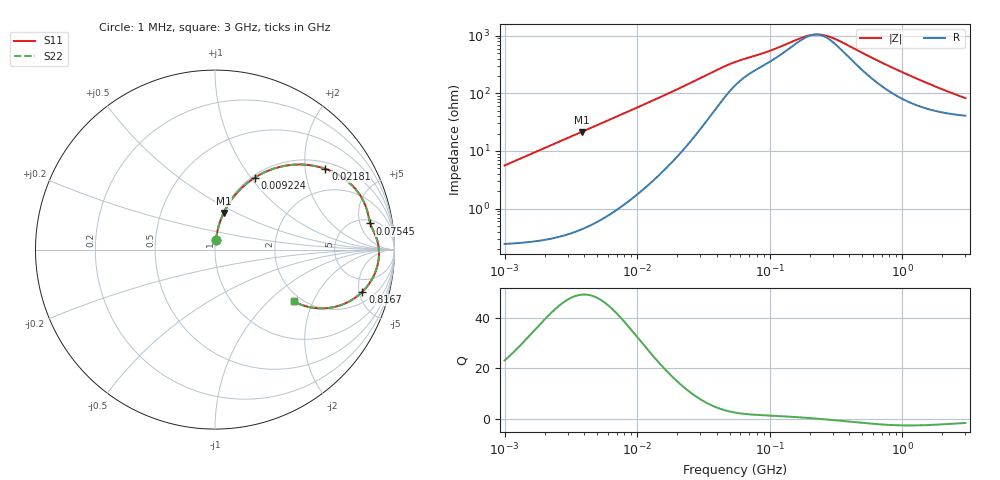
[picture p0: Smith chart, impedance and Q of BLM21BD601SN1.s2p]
! BLM21BD601SN1
# Hz S RI R 50
!Freq.(Hz) S11(Real) S11(Imag) S21(Real) S21(Imag) S12(Real) S12(Imag) S22(Real) S22(Imag)
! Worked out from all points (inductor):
!   401 points, 1 MHz to 3 GHz, reference 50 ohm
!   read as one part in series: L = 893 nH near 1.041 MHz
!   highest Q = 49.1 at 3.823 MHz (marker M1), where L = 894 nH
!   self-resonance near 220.5 MHz
!   S11 on the Smith chart (normalised r, x): 1 MHz: 1.00, +0.11; 9.224 MHz: 1.03, +1.04; 21.81 MHz: 1.20, +2.57; 75.45 MHz: 5.84, +7.39; 816.7 MHz: 3.10, -5.39; 3 GHz: 1.82, -1.44
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1000000  0.00555 0.0556  0.9945 -0.0556  0.9945 -0.0556  0.00555 0.0556
2055611  0.0159 0.1132  0.9841 -0.1132  0.9841 -0.1132  0.0159 0.1132
3823119  0.0479 0.2036  0.9521 -0.2036  0.9521 -0.2036  0.0479 0.2036
6180806  0.1135 0.3062  0.8865 -0.3062  0.8865 -0.3062  0.1135 0.3062
9223615  0.221 0.4007  0.779 -0.4007  0.779 -0.4007  0.221 0.4007
1.461624e7  0.4172 0.471  0.5828 -0.471  0.5828 -0.471  0.4172 0.471
2.181181e7  0.6154 0.4496  0.3846 -0.4496  0.3846 -0.4496  0.6154 0.4496
3.456417e7  0.787 0.3323  0.213 -0.3323  0.213 -0.3323  0.787 0.3323
5.477226e7  0.8516 0.2018  0.1484 -0.2018  0.1484 -0.2018  0.8516 0.2018
7.544761e7  0.865 0.1459  0.135 -0.1459  0.135 -0.1459  0.865 0.1459
1.060286e8  0.8838 0.1027  0.1162 -0.1027  0.1162 -0.1027  0.8838 0.1027
1.748812e8  0.908 0.0343  0.092 -0.0343  0.092 -0.0343  0.908 0.0343
2.094008e8  0.9122 0.0078  0.0878 -0.0078  0.0878 -0.0078  0.9122 0.0078
2.457655e8  0.9137 -0.0166  0.0863 0.0166  0.0863 0.0166  0.9137 -0.0166
2.942768e8  0.9126 -0.0451  0.0874 0.0451  0.0874 0.0451  0.9126 -0.0451
5.051982e8  0.8872 -0.1405  0.1128 0.1405  0.1128 0.1405  0.8872 -0.1405
8.005644e8  0.8249 -0.2311  0.1751 0.2311  0.1751 0.2311  0.8249 -0.2311
8.167498e8  0.821 -0.235  0.179 0.235  0.179 0.235  0.821 -0.235
1.194682e9  0.7273 -0.2989  0.2727 0.2989  0.2727 0.2989  0.7273 -0.2989
1.613037e9  0.6314 -0.3254  0.3686 0.3254  0.3686 0.3254  0.6314 -0.3254
2.134733e9  0.5374 -0.3226  0.4626 0.3226  0.4626 0.3226  0.5374 -0.3226
3e9  0.4374 -0.2876  0.5626 0.2876  0.5626 0.2876  0.4374 -0.2876
